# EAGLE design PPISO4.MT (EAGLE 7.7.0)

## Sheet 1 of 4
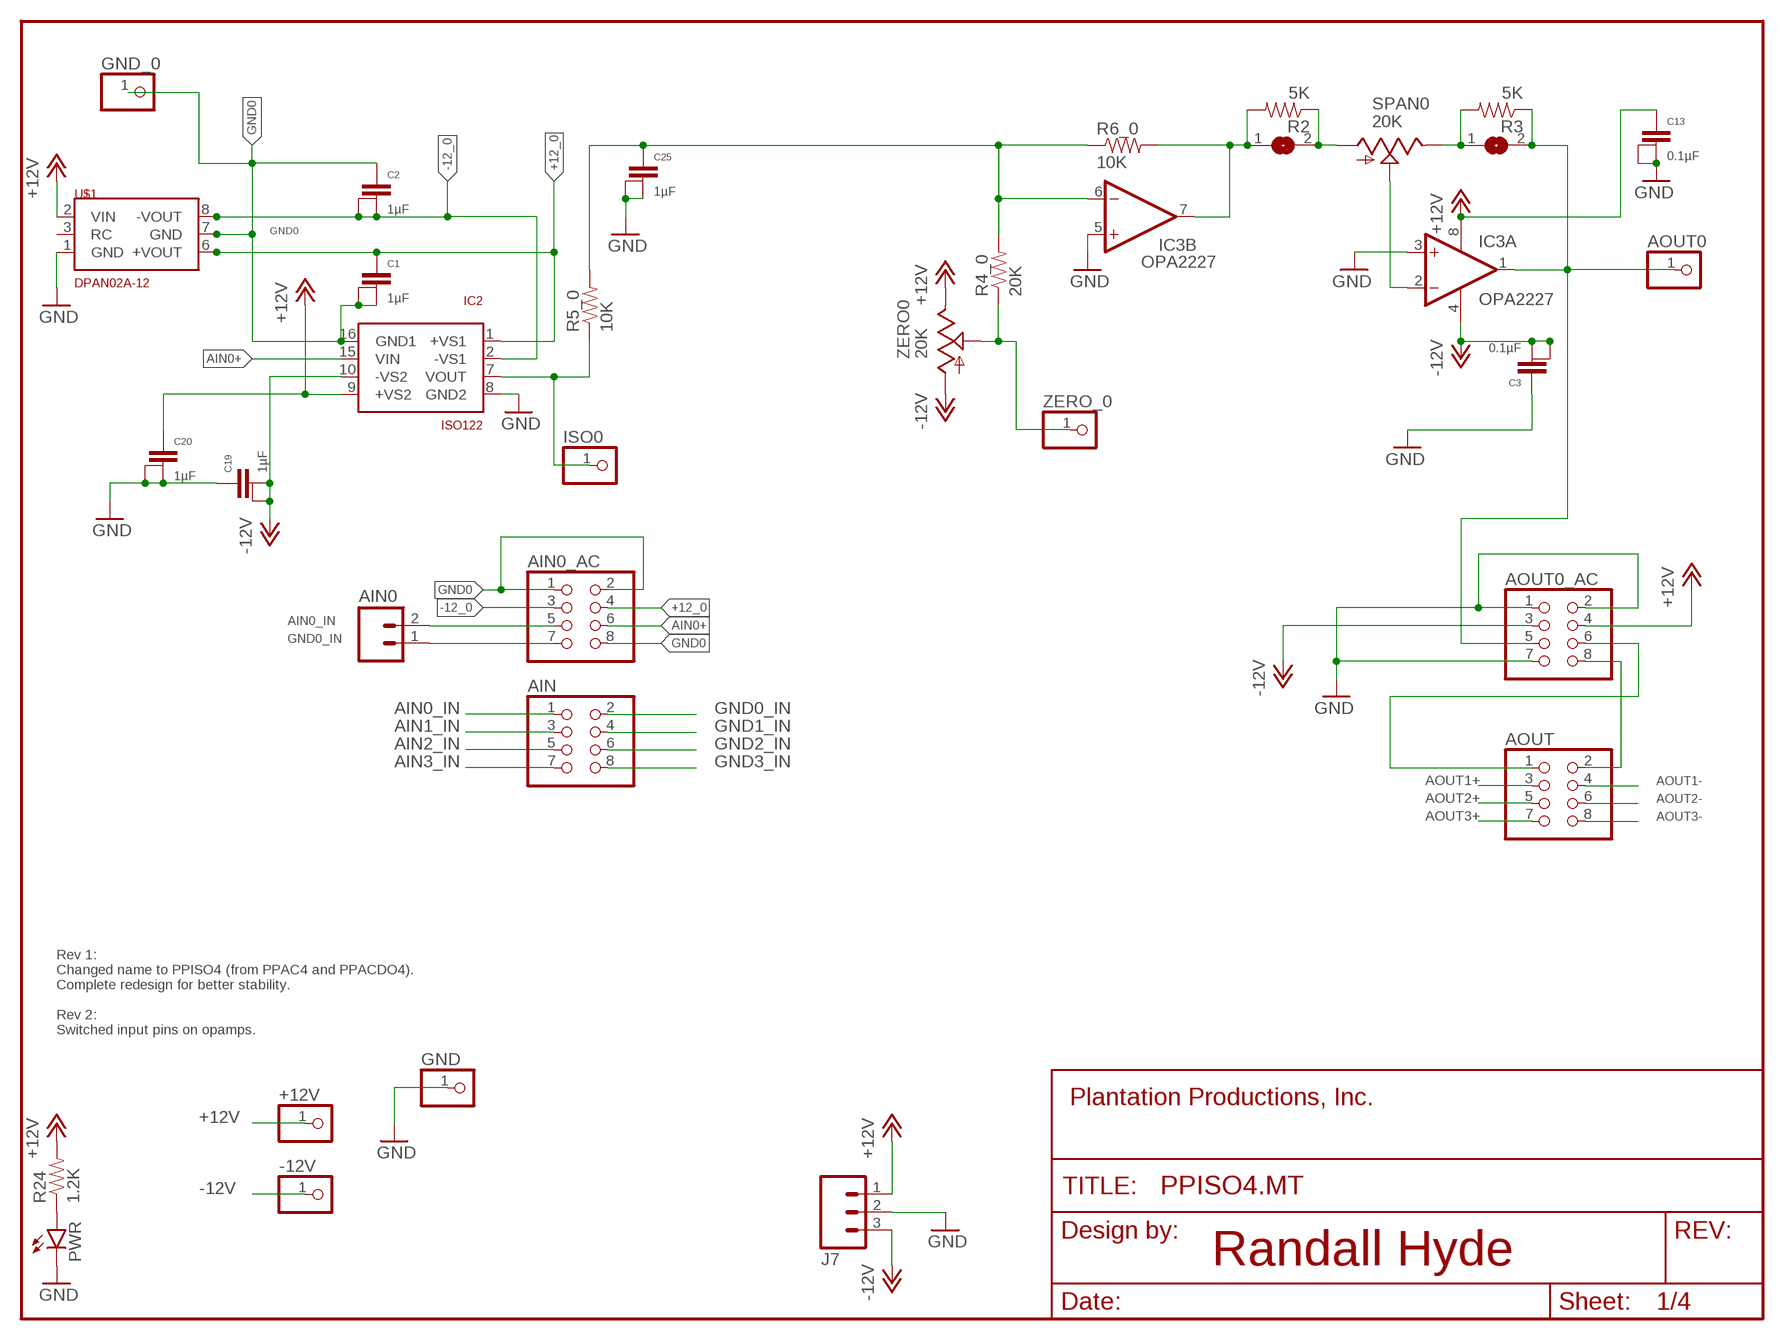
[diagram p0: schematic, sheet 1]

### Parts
+12V  PINHD-1X1  [1X01]
-12V  PINHD-1X1  [1X01]
AIN  PINHD-2X4  [2X04]
AIN0  M025MM  [SCREWTERMINAL-5MM-2]
AIN0_AC  PINHD-2X4  [2X04]
AOUT  PINHD-2X4  [2X04]
AOUT0  PINHD-1X1  [1X01]
AOUT0_AC  PINHD-2X4  [2X04]
C1  1µF  CAPACITOR  [1+2CAP]
C2  1µF  CAPACITOR  [1+2CAP]
C3  0.1µF  CAPACITOR  [1+2CAP]
C13  0.1µF  CAPACITOR  [1+2CAP]
C19  1µF  CAPACITOR  [1+2CAP]
C20  1µF  CAPACITOR  [1+2CAP]
C25  1µF  CAPACITOR  [1+2CAP]
FRAME1  FRAME-LETTERNO_PACKAGE  [DUMMY]
GND  PINHD-1X1  [1X01]
GND_0  PINHD-1X1  [1X01]
IC2  ISO122  [DIL16-8]
IC3  OPA2227  OPA2227N  [DIL08]
ISO0  PINHD-1X1  [1X01]
J7  M03-SCREW-5MM  [SCREWTERMINAL-5MM-3]
PWR  LED5MM  [LED5MM]
R2  5K  10OHM-1/4W-5%(PTH)  [AXIAL-0.3]
R3  5K  10OHM-1/4W-5%(PTH)  [AXIAL-0.3]
R4_0  20K  10OHM-1/4W-5%(PTH)  [AXIAL-0.3]
R5_0  10K  10OHM-1/4W-5%(PTH)  [AXIAL-0.3]
R6_0  10K  10OHM-1/4W-5%(PTH)  [AXIAL-0.3]
R24  1.2K  1KOHM-1/4W-1%(PTH)  [AXIAL-0.3]
SJ3  SOLDERJUMPERCLOSED  [SOLDERJUMPER_CLOSEDWIRE]
SJ4  SOLDERJUMPERCLOSED  [SOLDERJUMPER_CLOSEDWIRE]
SPAN0  20K  MULTIPOT  [B64WY]
U$1  DPAN02E-12  [DPAN-02E-12]
ZERO0  20K  MULTIPOT  [B64WY]
ZERO_0  PINHD-1X1  [1X01]

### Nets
+12_0 [RelayConn]: AIN0_AC.4 C1.1 IC2.1(+VS1) U$1.6(+VOUT)
+12V [RelayConn]: +12V.1 AOUT0_AC.4 C13.1 C20.1 IC2.9(+VS2) IC3.8(P:V+) J7.1 R24.P$2 U$1.2(VIN) ZERO0.E ZERO0.E1(E) ; also sheet 2,3,4
+12V3: R3.P$2 SJ4.1 SPAN0.E SPAN0.E1(E)
-12_0 [RelayConn]: AIN0_AC.3 C2.2@1 C2.2@2 IC2.2(-VS1) U$1.8(-VOUT)
-12V [RelayConn]: -12V.1 AOUT0_AC.3 C3.2@1 C3.2@2 C19.2@1 C19.2@2 IC2.10(-VS2) IC3.4(P:V-) J7.3 ZERO0.A ; also sheet 2,3,4
AIN0+: AIN0_AC.6 IC2.15(VIN)
AIN0_IN: AIN0.2 AIN0_AC.5 AIN.1
AIN1_IN: AIN.3 ; also sheet 2
AIN2_IN: AIN.5 ; also sheet 3
AIN3_IN: AIN.7 ; also sheet 4
AOUT0: AOUT0.1 AOUT0_AC.5 IC3.1(A:OUT) R3.P$1 SJ4.2
AOUT0+: AOUT0_AC.6 AOUT.1
AOUT0-: AOUT0_AC.8 AOUT.2
AOUT1+: AOUT.3 ; also sheet 2
AOUT1-: AOUT.4 ; also sheet 2
AOUT2+: AOUT.5 ; also sheet 3
AOUT2-: AOUT.6 ; also sheet 3
AOUT3+: AOUT.7 ; also sheet 4
AOUT3-: AOUT.8
GND [Ground]: AOUT0_AC.1 AOUT0_AC.2 AOUT0_AC.7 C3.1 C13.2@1 C13.2@2 C19.1 C20.2@1 C20.2@2 C25.2@1 C25.2@2 GND.1 IC2.8(GND2) IC3.3(A:+IN) IC3.5(B:+IN) J7.2 PWR.K(C) U$1.1(GND) ; also sheet 2,3,4
GND0: AIN0_AC.1 AIN0_AC.2 AIN0_AC.8 C1.2@1 C1.2@2 C2.1 GND_0.1 IC2.16(GND1) U$1.7(GND)
GND0_IN: AIN0.1 AIN0_AC.7 AIN.2
GND1_IN: AIN.4 ; also sheet 2
GND2_IN: AIN.6 ; also sheet 3
GND3_IN: AIN.8 ; also sheet 4
IC1_9: IC3.7(B:OUT) R2.P$2 R6_0.P$2 SJ3.1
N$4: IC3.2(A:-IN) SPAN0.A1(S) SPAN0.S SPAN0.S1(S)
N$6: R4_0.P$1 ZERO0.A1(S) ZERO0.S ZERO0.S1(S) ZERO_0.1
N$8: IC2.7(VOUT) ISO0.1 R5_0.P$1
N$26: PWR.A R24.P$1
N$43: C25.1 IC3.6(B:-IN) R4_0.P$2 R5_0.P$2 R6_0.P$1
N$58: R2.P$1 SJ3.2 SPAN0.A
Unconnected: U$1.3(RC)

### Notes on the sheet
- Rev 1:
  Changed name to PPISO4 (from PPAC4 and PPACDO4).
  Complete redesign for better stability.
  
  Rev 2:
  Switched input pins on opamps.
- Randall Hyde

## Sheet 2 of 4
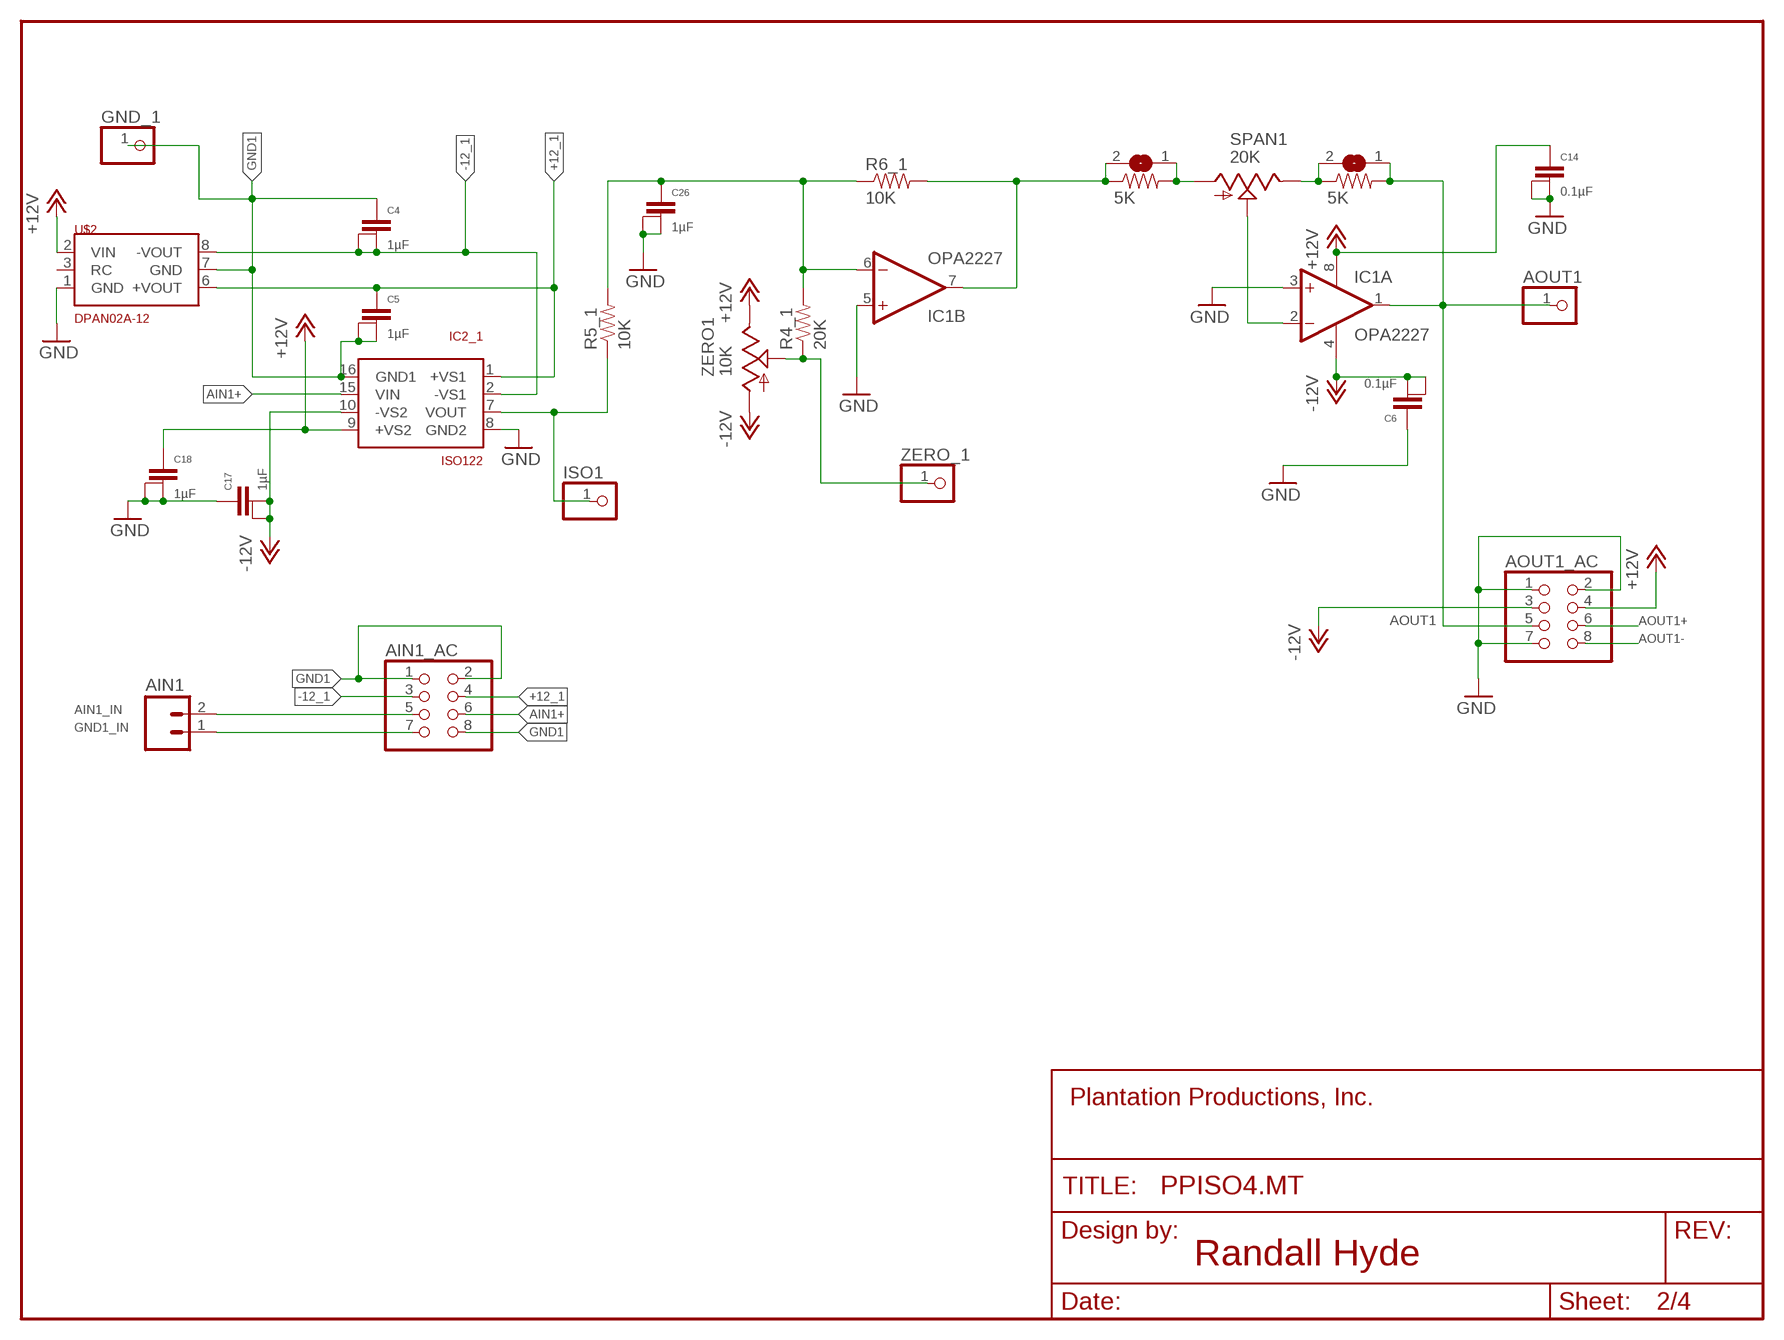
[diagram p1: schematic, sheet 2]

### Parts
AIN1  M025MM  [SCREWTERMINAL-5MM-2]
AIN1_AC  PINHD-2X4  [2X04]
AOUT1  PINHD-1X1  [1X01]
AOUT1_AC  PINHD-2X4  [2X04]
C4  1µF  CAPACITOR  [1+2CAP]
C5  1µF  CAPACITOR  [1+2CAP]
C6  0.1µF  CAPACITOR  [1+2CAP]
C14  0.1µF  CAPACITOR  [1+2CAP]
C17  1µF  CAPACITOR  [1+2CAP]
C18  1µF  CAPACITOR  [1+2CAP]
C26  1µF  CAPACITOR  [1+2CAP]
FRAME2  FRAME-LETTERNO_PACKAGE  [DUMMY]
GND_1  PINHD-1X1  [1X01]
IC1  OPA2227  OPA2227N  [DIL08]
IC2_1  ISO122  [DIL16-8]
ISO1  PINHD-1X1  [1X01]
R4_1  20K  10OHM-1/4W-5%(PTH)  [AXIAL-0.3]
R5_1  10K  10OHM-1/4W-5%(PTH)  [AXIAL-0.3]
R6  5K  10OHM-1/4W-5%(PTH)  [AXIAL-0.3]
R6_1  10K  10OHM-1/4W-5%(PTH)  [AXIAL-0.3]
R11  5K  10OHM-1/4W-5%(PTH)  [AXIAL-0.3]
SJ7  SOLDERJUMPERCLOSED  [SOLDERJUMPER_CLOSEDWIRE]
SJ12  SOLDERJUMPERCLOSED  [SOLDERJUMPER_CLOSEDWIRE]
SPAN1  20K  MULTIPOT  [B64WY]
U$2  DPAN02E-12  [DPAN-02E-12]
ZERO1  10K  MULTIPOT  [B64WY]
ZERO_1  PINHD-1X1  [1X01]

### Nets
+12_1 [RelayConn]: AIN1_AC.4 C5.1 IC2_1.1(+VS1) U$2.6(+VOUT)
+12V [RelayConn]: AOUT1_AC.4 C14.1 C18.1 IC1.8(P:V+) IC2_1.9(+VS2) U$2.2(VIN) ZERO1.E ZERO1.E1(E) ; also sheet 1,3,4
-12_1 [RelayConn]: AIN1_AC.3 C4.2@1 C4.2@2 IC2_1.2(-VS1) U$2.8(-VOUT)
-12V [RelayConn]: AOUT1_AC.3 C6.2@1 C6.2@2 C17.2@1 C17.2@2 IC1.4(P:V-) IC2_1.10(-VS2) ZERO1.A ; also sheet 1,3,4
AIN1+: AIN1_AC.6 IC2_1.15(VIN)
AIN1_IN: AIN1.2 AIN1_AC.5 ; also sheet 1
AOUT1: AOUT1.1 AOUT1_AC.5 IC1.1(A:OUT) R6.P$2 SJ7.1
AOUT1+: AOUT1_AC.6 ; also sheet 1
AOUT1-: AOUT1_AC.8 ; also sheet 1
GND [Ground]: AOUT1_AC.1 AOUT1_AC.2 AOUT1_AC.7 C6.1 C14.2@1 C14.2@2 C17.1 C18.2@1 C18.2@2 C26.2@1 C26.2@2 IC1.3(A:+IN) IC1.5(B:+IN) IC2_1.8(GND2) U$2.1(GND) ; also sheet 1,3,4
GND1: AIN1_AC.1 AIN1_AC.2 AIN1_AC.8 C4.1 C5.2@1 C5.2@2 GND_1.1 IC2_1.16(GND1) U$2.7(GND)
GND1_IN: AIN1.1 AIN1_AC.7 ; also sheet 1
IC2_8: IC1.7(B:OUT) R6_1.P$2 R11.P$1 SJ12.2
N$1: C26.1 IC1.6(B:-IN) R4_1.P$2 R5_1.P$2 R6_1.P$1
N$3: R6.P$1 SJ7.2 SPAN1.E SPAN1.E1(E)
N$19: IC1.2(A:-IN) SPAN1.A1(S) SPAN1.S SPAN1.S1(S)
N$22: IC2_1.7(VOUT) ISO1.1 R5_1.P$1
N$23: R4_1.P$1 ZERO1.A1(S) ZERO1.S ZERO1.S1(S) ZERO_1.1
SPAN1L: R11.P$2 SJ12.1 SPAN1.A
Unconnected: U$2.3(RC)

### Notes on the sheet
- Randall Hyde

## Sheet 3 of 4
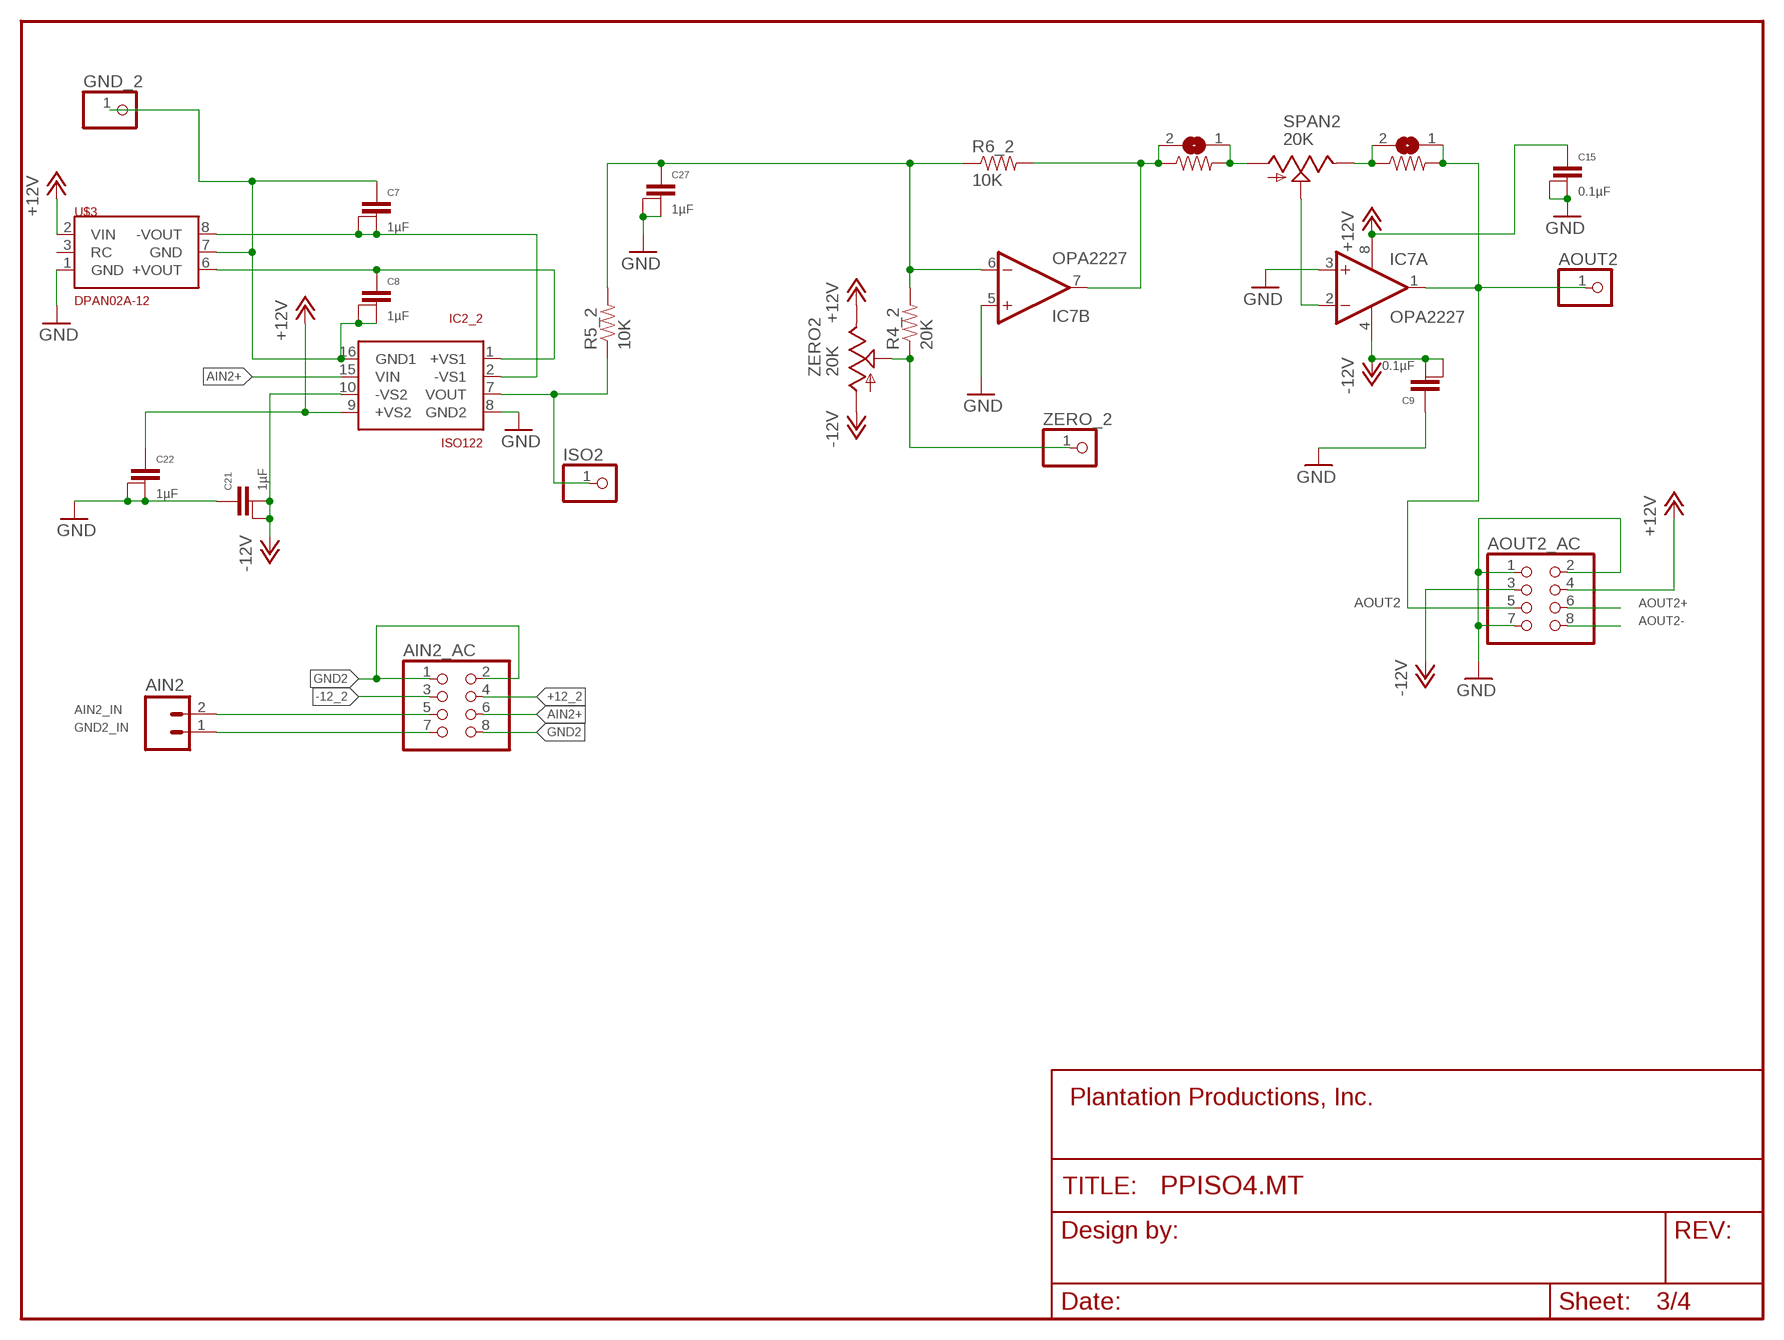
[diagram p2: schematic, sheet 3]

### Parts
AIN2  M025MM  [SCREWTERMINAL-5MM-2]
AIN2_AC  PINHD-2X4  [2X04]
AOUT2  PINHD-1X1  [1X01]
AOUT2_AC  PINHD-2X4  [2X04]
C7  1µF  CAPACITOR  [1+2CAP]
C8  1µF  CAPACITOR  [1+2CAP]
C9  0.1µF  CAPACITOR  [1+2CAP]
C15  0.1µF  CAPACITOR  [1+2CAP]
C21  1µF  CAPACITOR  [1+2CAP]
C22  1µF  CAPACITOR  [1+2CAP]
C27  1µF  CAPACITOR  [1+2CAP]
FRAME3  FRAME-LETTERNO_PACKAGE  [DUMMY]
GND_2  PINHD-1X1  [1X01]
IC2_2  ISO122  [DIL16-8]
IC7  OPA2227  OPA2227N  [DIL08]
ISO2  PINHD-1X1  [1X01]
R4_2  20K  10OHM-1/4W-5%(PTH)  [AXIAL-0.3]
R5_2  10K  10OHM-1/4W-5%(PTH)  [AXIAL-0.3]
R6_2  10K  10OHM-1/4W-5%(PTH)  [AXIAL-0.3]
R12  5K  10OHM-1/4W-5%(PTH)  [AXIAL-0.3]
R17  5K  10OHM-1/4W-5%(PTH)  [AXIAL-0.3]
SJ13  SOLDERJUMPERCLOSED  [SOLDERJUMPER_CLOSEDWIRE]
SJ18  SOLDERJUMPERCLOSED  [SOLDERJUMPER_CLOSEDWIRE]
SPAN2  20K  MULTIPOT  [B64WY]
U$3  DPAN02E-12  [DPAN-02E-12]
ZERO2  20K  MULTIPOT  [B64WY]
ZERO_2  PINHD-1X1  [1X01]

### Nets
+12_2 [RelayConn]: AIN2_AC.4 C8.1 IC2_2.1(+VS1) U$3.6(+VOUT)
+12V [RelayConn]: AOUT2_AC.4 C15.1 C22.1 IC2_2.9(+VS2) IC7.8(P:V+) U$3.2(VIN) ZERO2.E ZERO2.E1(E) ; also sheet 1,2,4
+12V10: R17.P$2 SJ18.1 SPAN2.A
-12_2 [RelayConn]: AIN2_AC.3 C7.2@1 C7.2@2 IC2_2.2(-VS1) U$3.8(-VOUT)
-12V [RelayConn]: AOUT2_AC.3 C9.2@1 C9.2@2 C21.2@1 C21.2@2 IC2_2.10(-VS2) IC7.4(P:V-) ZERO2.A ; also sheet 1,2,4
AIN2+: AIN2_AC.6 IC2_2.15(VIN)
AIN2_IN: AIN2.2 AIN2_AC.5 ; also sheet 1
AOUT2: AOUT2.1 AOUT2_AC.5 IC7.1(A:OUT) R12.P$2 SJ13.1
AOUT2+: AOUT2_AC.6 ; also sheet 1
AOUT2-: AOUT2_AC.8 ; also sheet 1
GND [Ground]: AOUT2_AC.1 AOUT2_AC.2 AOUT2_AC.7 C9.1 C15.2@1 C15.2@2 C21.1 C22.2@1 C22.2@2 C27.2@1 C27.2@2 IC2_2.8(GND2) IC7.3(A:+IN) IC7.5(B:+IN) U$3.1(GND) ; also sheet 1,2,4
GND2: AIN2_AC.1 AIN2_AC.2 AIN2_AC.8 C7.1 C8.2@1 C8.2@2 GND_2.1 IC2_2.16(GND1) U$3.7(GND)
GND2_IN: AIN2.1 AIN2_AC.7 ; also sheet 1
N$18: R12.P$1 SJ13.2 SPAN2.E SPAN2.E1(E)
N$34: IC2_2.7(VOUT) ISO2.1 R5_2.P$1
N$35: IC7.2(A:-IN) SPAN2.A1(S) SPAN2.S SPAN2.S1(S)
N$36: IC7.7(B:OUT) R6_2.P$2 R17.P$1 SJ18.2
N$40: R4_2.P$1 ZERO2.A1(S) ZERO2.S ZERO2.S1(S) ZERO_2.1
N$60: C27.1 IC7.6(B:-IN) R4_2.P$2 R5_2.P$2 R6_2.P$1
Unconnected: U$3.3(RC)

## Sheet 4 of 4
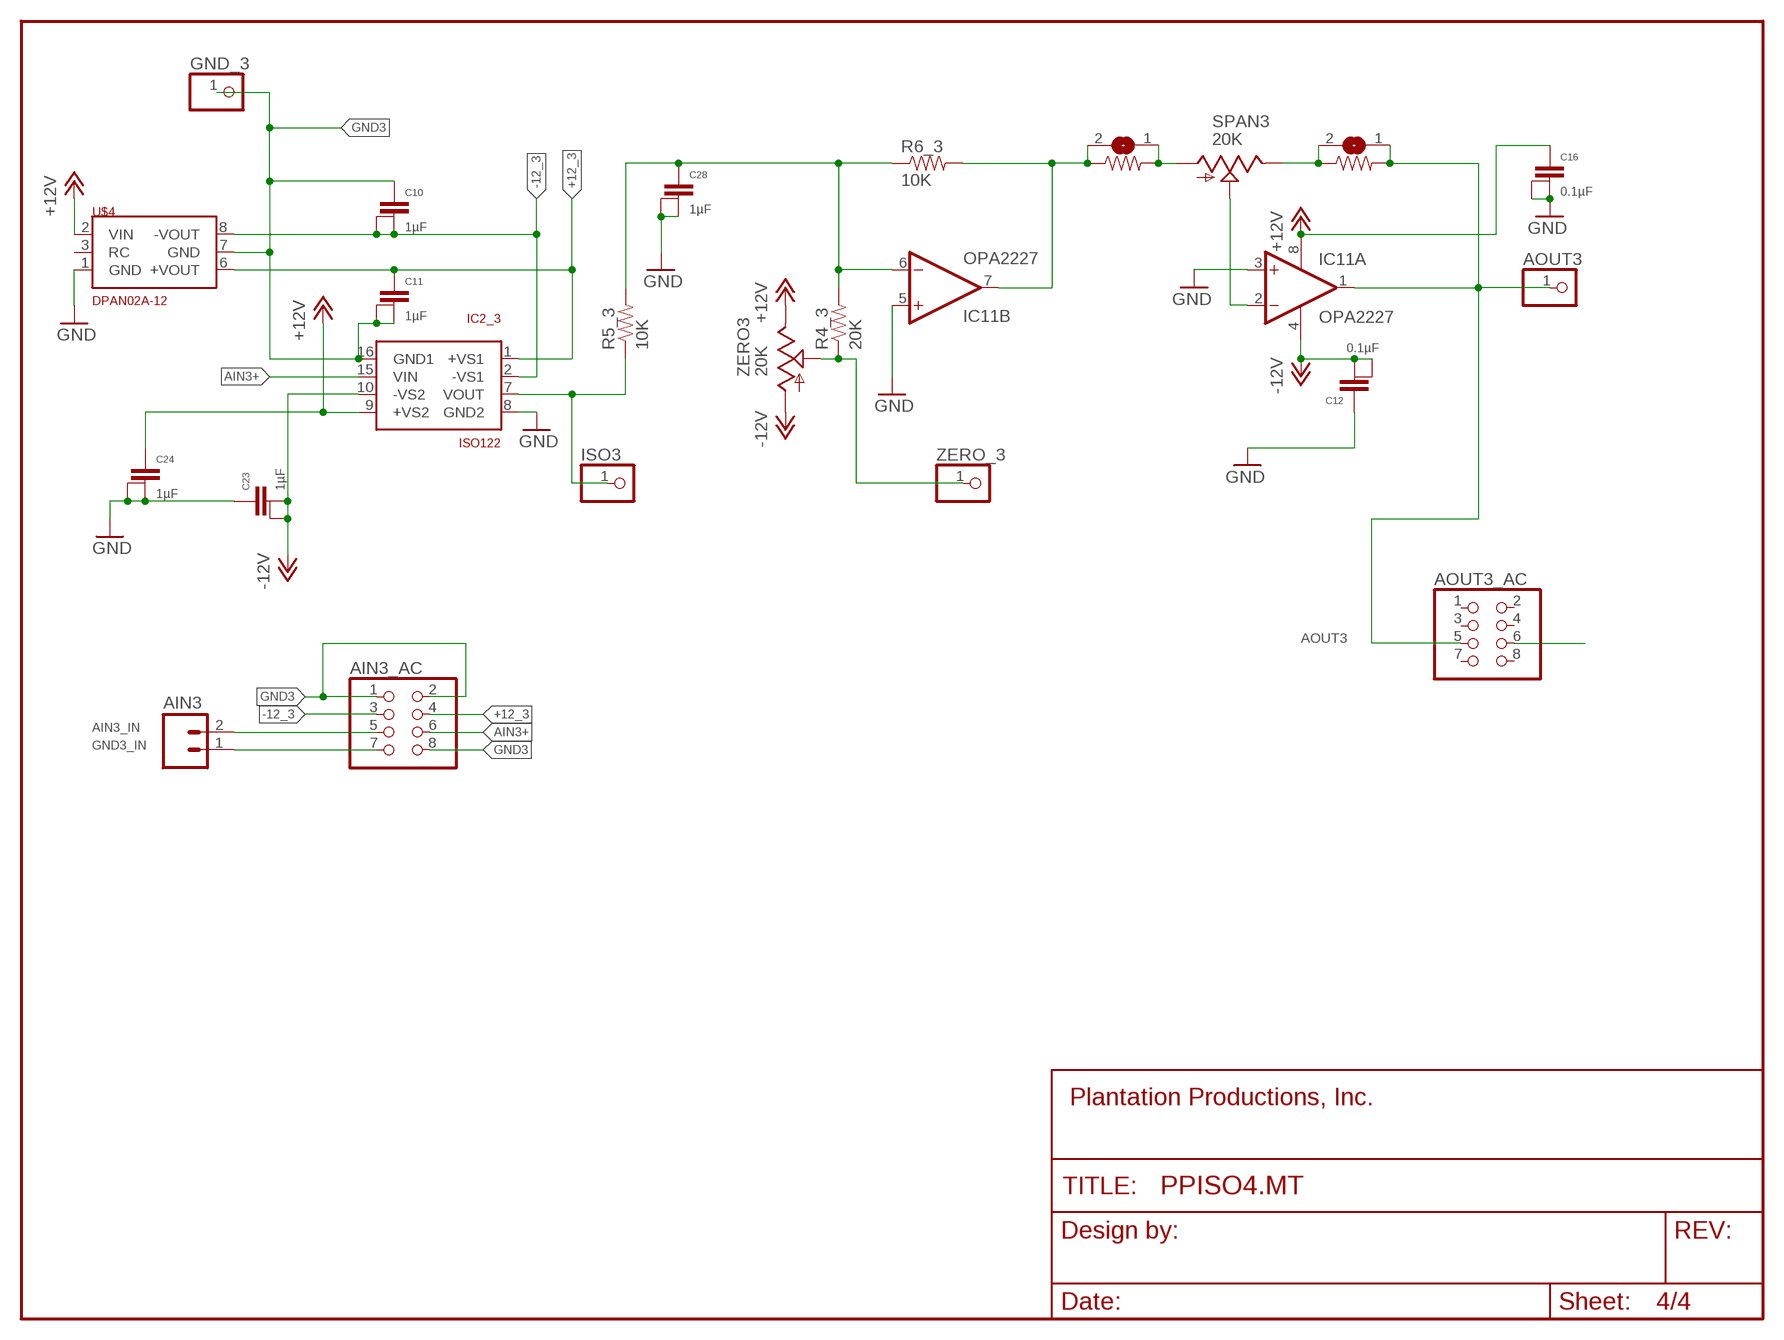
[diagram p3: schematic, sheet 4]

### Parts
AIN3  M025MM  [SCREWTERMINAL-5MM-2]
AIN3_AC  PINHD-2X4  [2X04]
AOUT3  PINHD-1X1  [1X01]
AOUT3_AC  PINHD-2X4  [2X04]
C10  1µF  CAPACITOR  [1+2CAP]
C11  1µF  CAPACITOR  [1+2CAP]
C12  0.1µF  CAPACITOR  [1+2CAP]
C16  0.1µF  CAPACITOR  [1+2CAP]
C23  1µF  CAPACITOR  [1+2CAP]
C24  1µF  CAPACITOR  [1+2CAP]
C28  1µF  CAPACITOR  [1+2CAP]
FRAME4  FRAME-LETTERNO_PACKAGE  [DUMMY]
GND_3  PINHD-1X1  [1X01]
IC2_3  ISO122  [DIL16-8]
IC11  OPA2227  OPA2227N  [DIL08]
ISO3  PINHD-1X1  [1X01]
R4_3  20K  10OHM-1/4W-5%(PTH)  [AXIAL-0.3]
R5_3  10K  10OHM-1/4W-5%(PTH)  [AXIAL-0.3]
R6_3  10K  10OHM-1/4W-5%(PTH)  [AXIAL-0.3]
R18  5K  10OHM-1/4W-5%(PTH)  [AXIAL-0.3]
R23  5K  10OHM-1/4W-5%(PTH)  [AXIAL-0.3]
SJ19  SOLDERJUMPERCLOSED  [SOLDERJUMPER_CLOSEDWIRE]
SJ24  SOLDERJUMPERCLOSED  [SOLDERJUMPER_CLOSEDWIRE]
SPAN3  20K  MULTIPOT  [B64WY]
U$4  DPAN02E-12  [DPAN-02E-12]
ZERO3  20K  MULTIPOT  [B64WY]
ZERO_3  PINHD-1X1  [1X01]

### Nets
+12_3 [RelayConn]: AIN3_AC.4 C11.1 IC2_3.1(+VS1) U$4.6(+VOUT)
+12V [RelayConn]: C16.1 C24.1 IC2_3.9(+VS2) IC11.8(P:V+) U$4.2(VIN) ZERO3.E ZERO3.E1(E) ; also sheet 1,2,3
+12V4: R18.P$2 SJ19.1 SPAN3.A
-12_3 [RelayConn]: AIN3_AC.3 C10.2@1 C10.2@2 IC2_3.2(-VS1) U$4.8(-VOUT)
-12V [RelayConn]: C12.2@1 C12.2@2 C23.2@1 C23.2@2 IC2_3.10(-VS2) IC11.4(P:V-) ZERO3.A ; also sheet 1,2,3
AIN3+: AIN3_AC.6 IC2_3.15(VIN)
AIN3_IN: AIN3.2 AIN3_AC.5 ; also sheet 1
AOUT3: AOUT3.1 AOUT3_AC.5 IC11.1(A:OUT) R23.P$2 SJ24.1
AOUT3+: AOUT3_AC.6 ; also sheet 1
GND [Ground]: C12.1 C16.2@1 C16.2@2 C23.1 C24.2@1 C24.2@2 C28.2@1 C28.2@2 IC2_3.8(GND2) IC11.3(A:+IN) IC11.5(B:+IN) U$4.1(GND) ; also sheet 1,2,3
GND3: AIN3_AC.1 AIN3_AC.2 AIN3_AC.8 C10.1 C11.2@1 C11.2@2 GND_3.1 IC2_3.16(GND1) U$4.7(GND)
GND3_IN: AIN3.1 AIN3_AC.7 ; also sheet 1
N$17: IC11.2(A:-IN) SPAN3.A1(S) SPAN3.S SPAN3.S1(S)
N$27: IC11.7(B:OUT) R6_3.P$2 R18.P$1 SJ19.2
N$37: R23.P$1 SJ24.2 SPAN3.E SPAN3.E1(E)
N$39: C28.1 IC11.6(B:-IN) R4_3.P$2 R5_3.P$2 R6_3.P$1
N$55: IC2_3.7(VOUT) ISO3.1 R5_3.P$1
N$56: R4_3.P$1 ZERO3.A1(S) ZERO3.S ZERO3.S1(S) ZERO_3.1
Unconnected: AOUT3_AC.1 AOUT3_AC.2 AOUT3_AC.3 AOUT3_AC.4 AOUT3_AC.7 AOUT3_AC.8 U$4.3(RC)

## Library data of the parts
+12V -12V AOUT0 AOUT1-AOUT3 GND GND_0 GND_1-GND_3 ISO0 ISO1-ISO3 ZERO_0 ZERO_1-ZERO_3 = pinhead:PINHD-1X1: PIN HEADER
AIN AIN0_AC AIN1_AC AIN2_AC AIN3_AC AOUT AOUT0_AC AOUT1_AC AOUT2_AC AOUT3_AC = pinhead:PINHD-2X4: PIN HEADER
AIN0 AIN1-AIN3 = SparkFun-Connectors:M02: Standard 2-pin 0.1" header. Use with; STOREFRONT_ID: PRT-08432
C1-C28 = PlantProd:CAPACITOR: Capacitor with three terminals to support multiple capacitor sizes.
FRAME1-FRAME4 = SparkFun-Aesthetics:FRAME-LETTER: Schematic Frame; DESIGNER: Nobody; VERSION: v01
IC1 IC3 IC7 IC11 = linear:OPA222*: High Precision, Low Noise OPERATIONAL AMPLIFIERS Source: http://focus.ti.com/lit/ds/symlink/opa227.pdf
IC2 IC2_1-IC2_3 = PlantProd:ISO122: ISO122 - single channel isolation amplifier
J7 = SparkFun-Connectors:M03: Header 3 Standard 3-pin 0.1" header. Use with straight break away headers (SKU : PRT-00116), right angle break away headers (PRT-00553), swiss pins (PRT-00743), machine pins (PRT-00117), and female headers (PRT-00115). Molex polarized connector foot print use with SKU : PRT-08232 with associated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; STOREFRONT_ID: PRT-08433
PWR = SparkFun-LED:LED: LEDs
R2 R3 R4_0 R4_1-R4_3 R5_0 R5_1-R5_3 R6 R6_0 R6_1-R6_3 R11 R12 R17 R18 R23 = SparkFun-Resistors:10OHM-1/4W-5%(PTH): RES-10698; PROD_ID: RES-10698; VALUE: 10
R24 = SparkFun-Resistors:1KOHM-1/4W-1%(PTH): RES-12182; PROD_ID: RES-12182; VALUE: 1K
SJ3 SJ4 SJ7 SJ12 SJ13 SJ18 SJ19 SJ24 = microbuilder:SOLDERJUMPER: SMD Solder JUMPER
SPAN0 SPAN1-SPAN3 ZERO0 ZERO1-ZERO3 = PlantProd:MULTIPOT
U$1-U$4 = PlantProd:DPAN02E-12

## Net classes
1 Ground: width 0.762 mm, drill 1 mm, clearance 0.102 mm
2 RelayConn: width 1.016 mm, drill 0.025 mm, clearance 0.508 mm
3 HiCurSignal: width 1.016 mm, drill 0.025 mm, clearance 1.016 mm

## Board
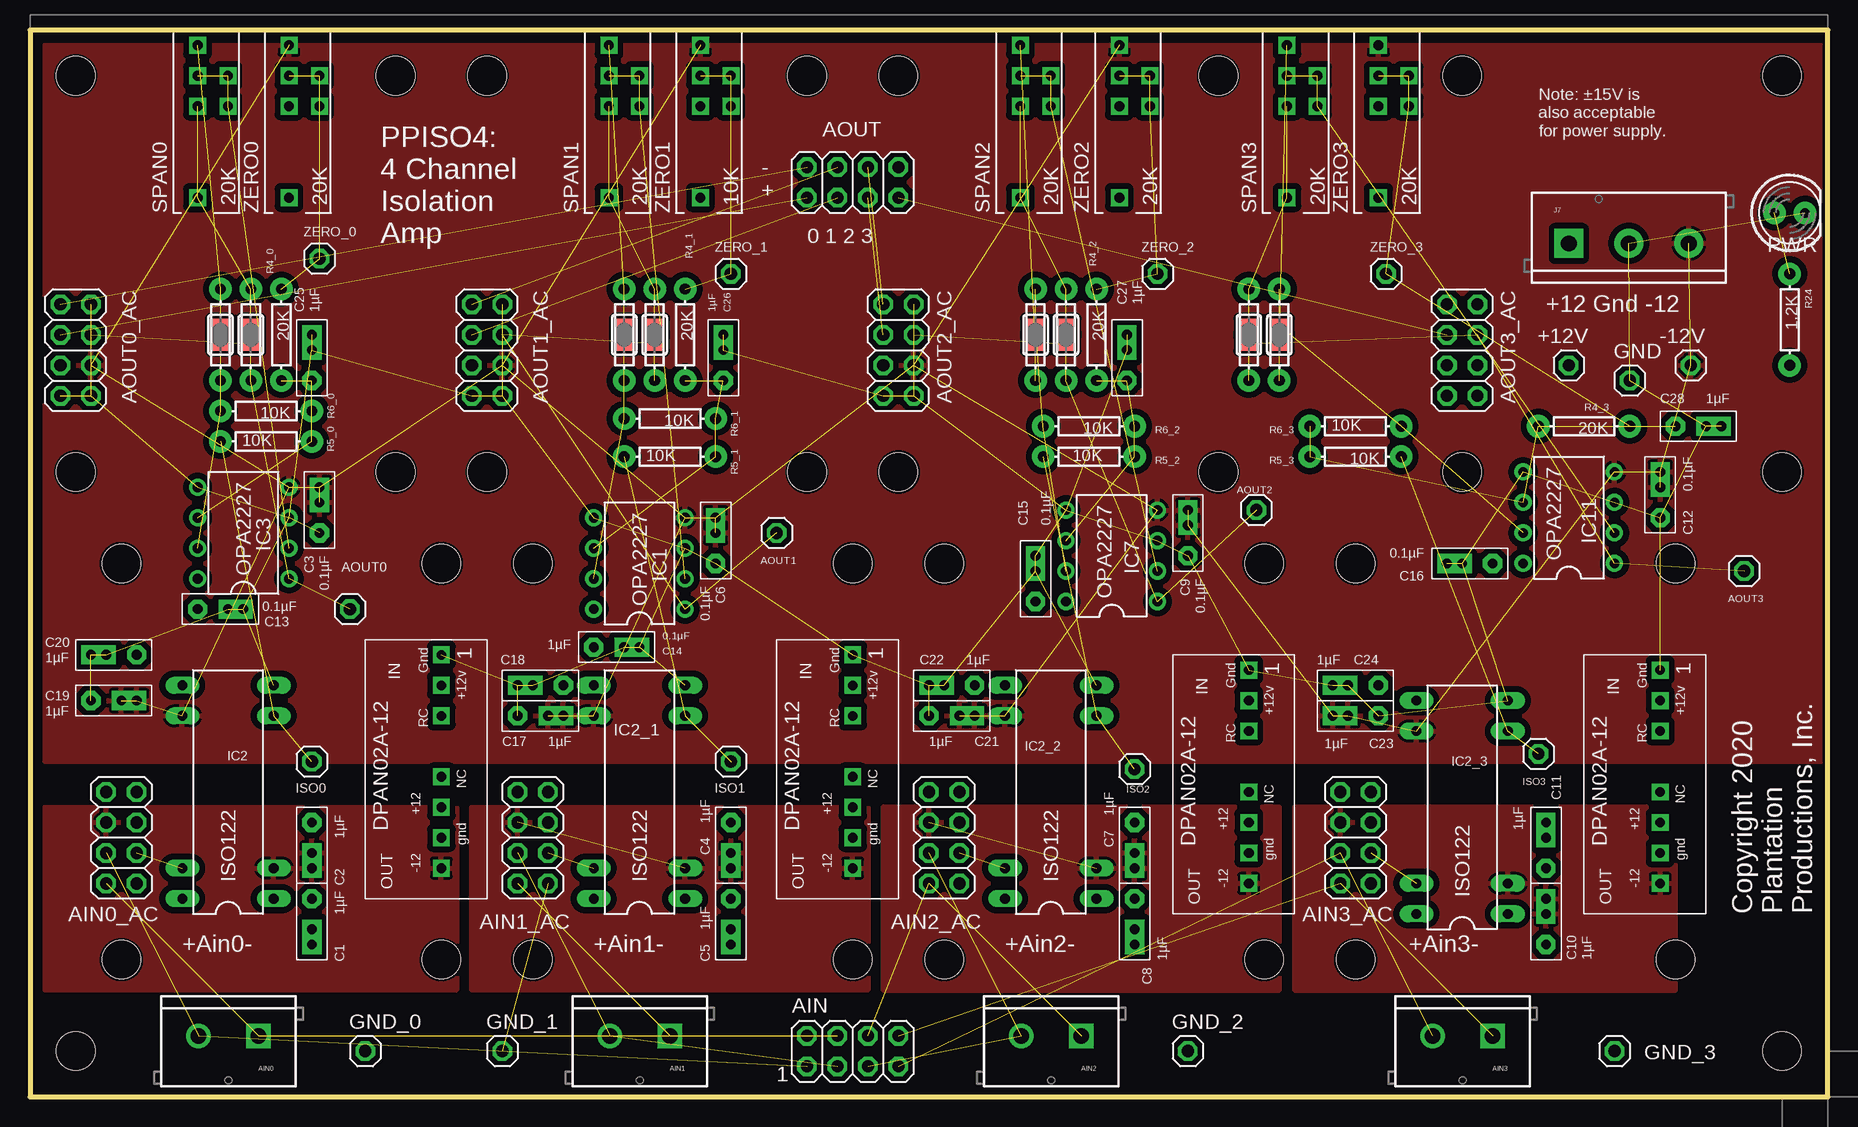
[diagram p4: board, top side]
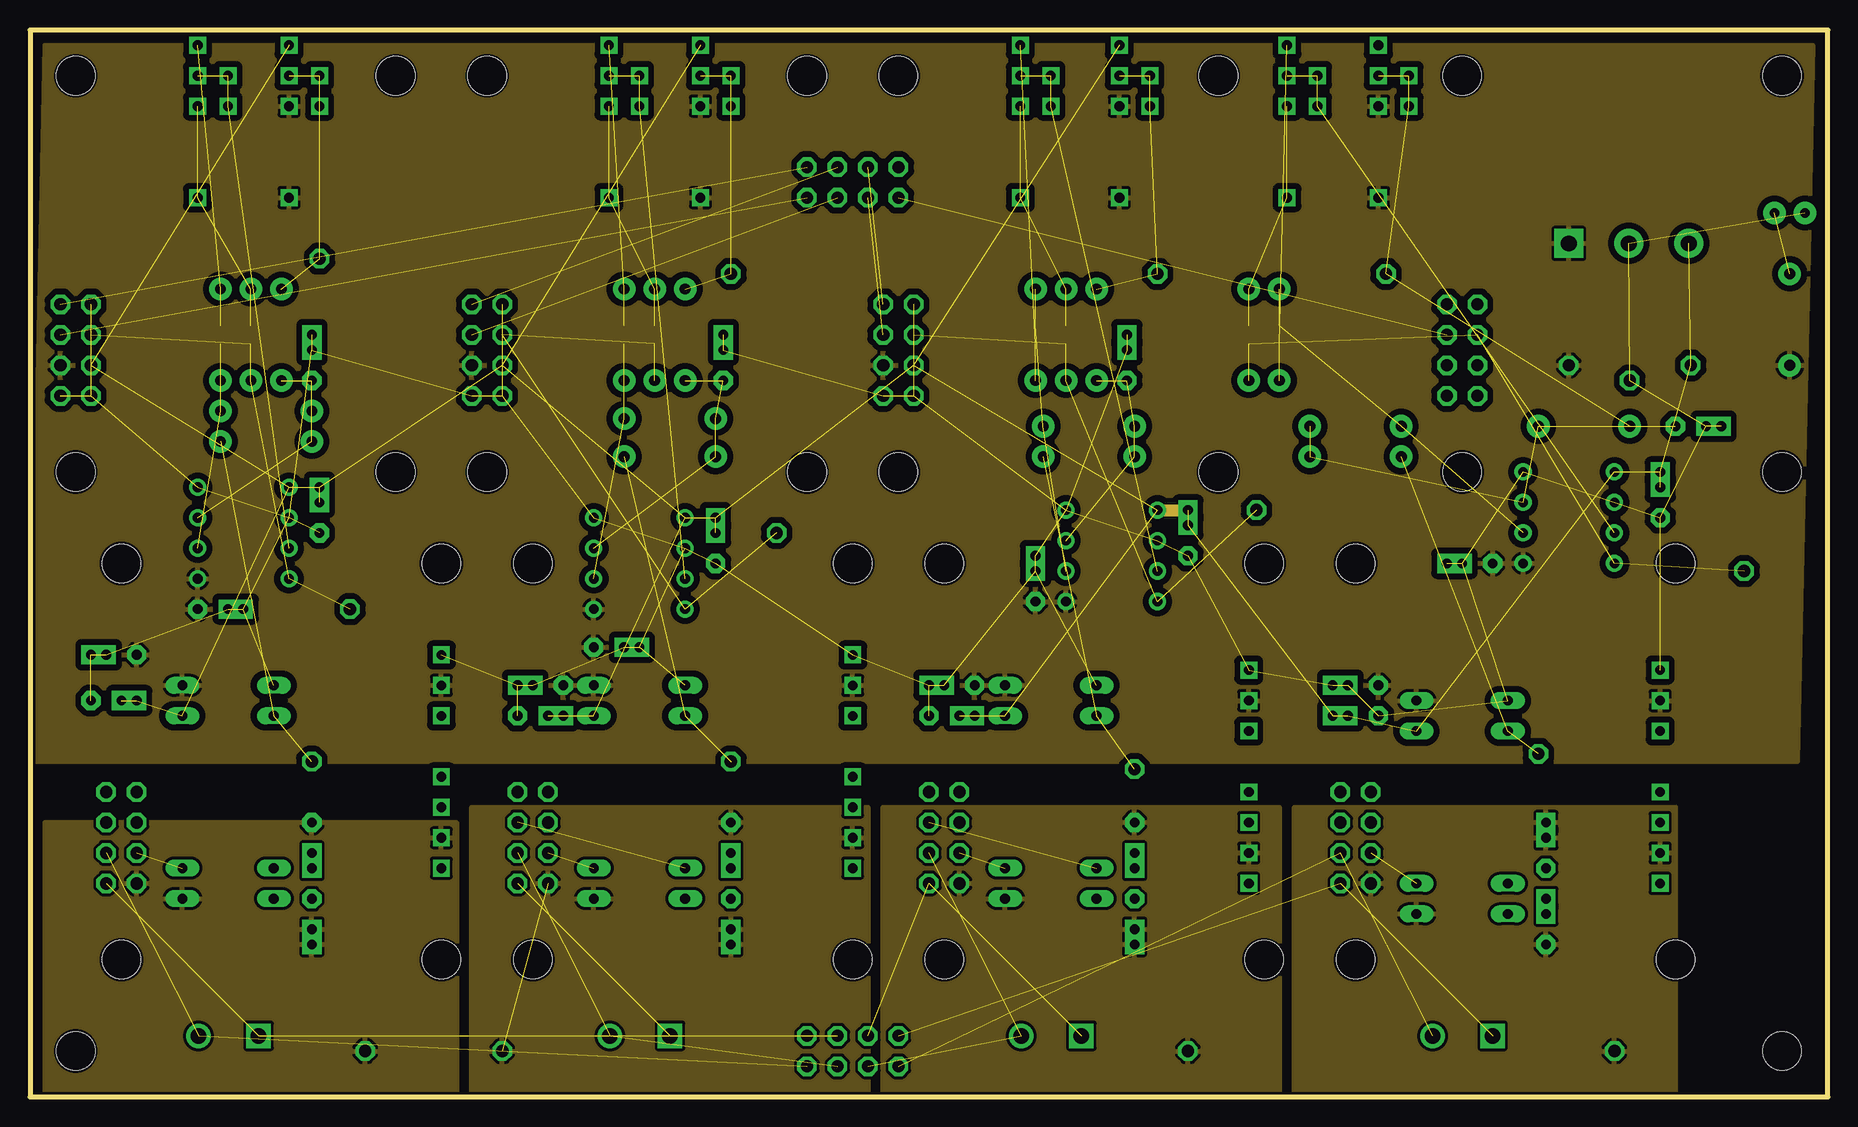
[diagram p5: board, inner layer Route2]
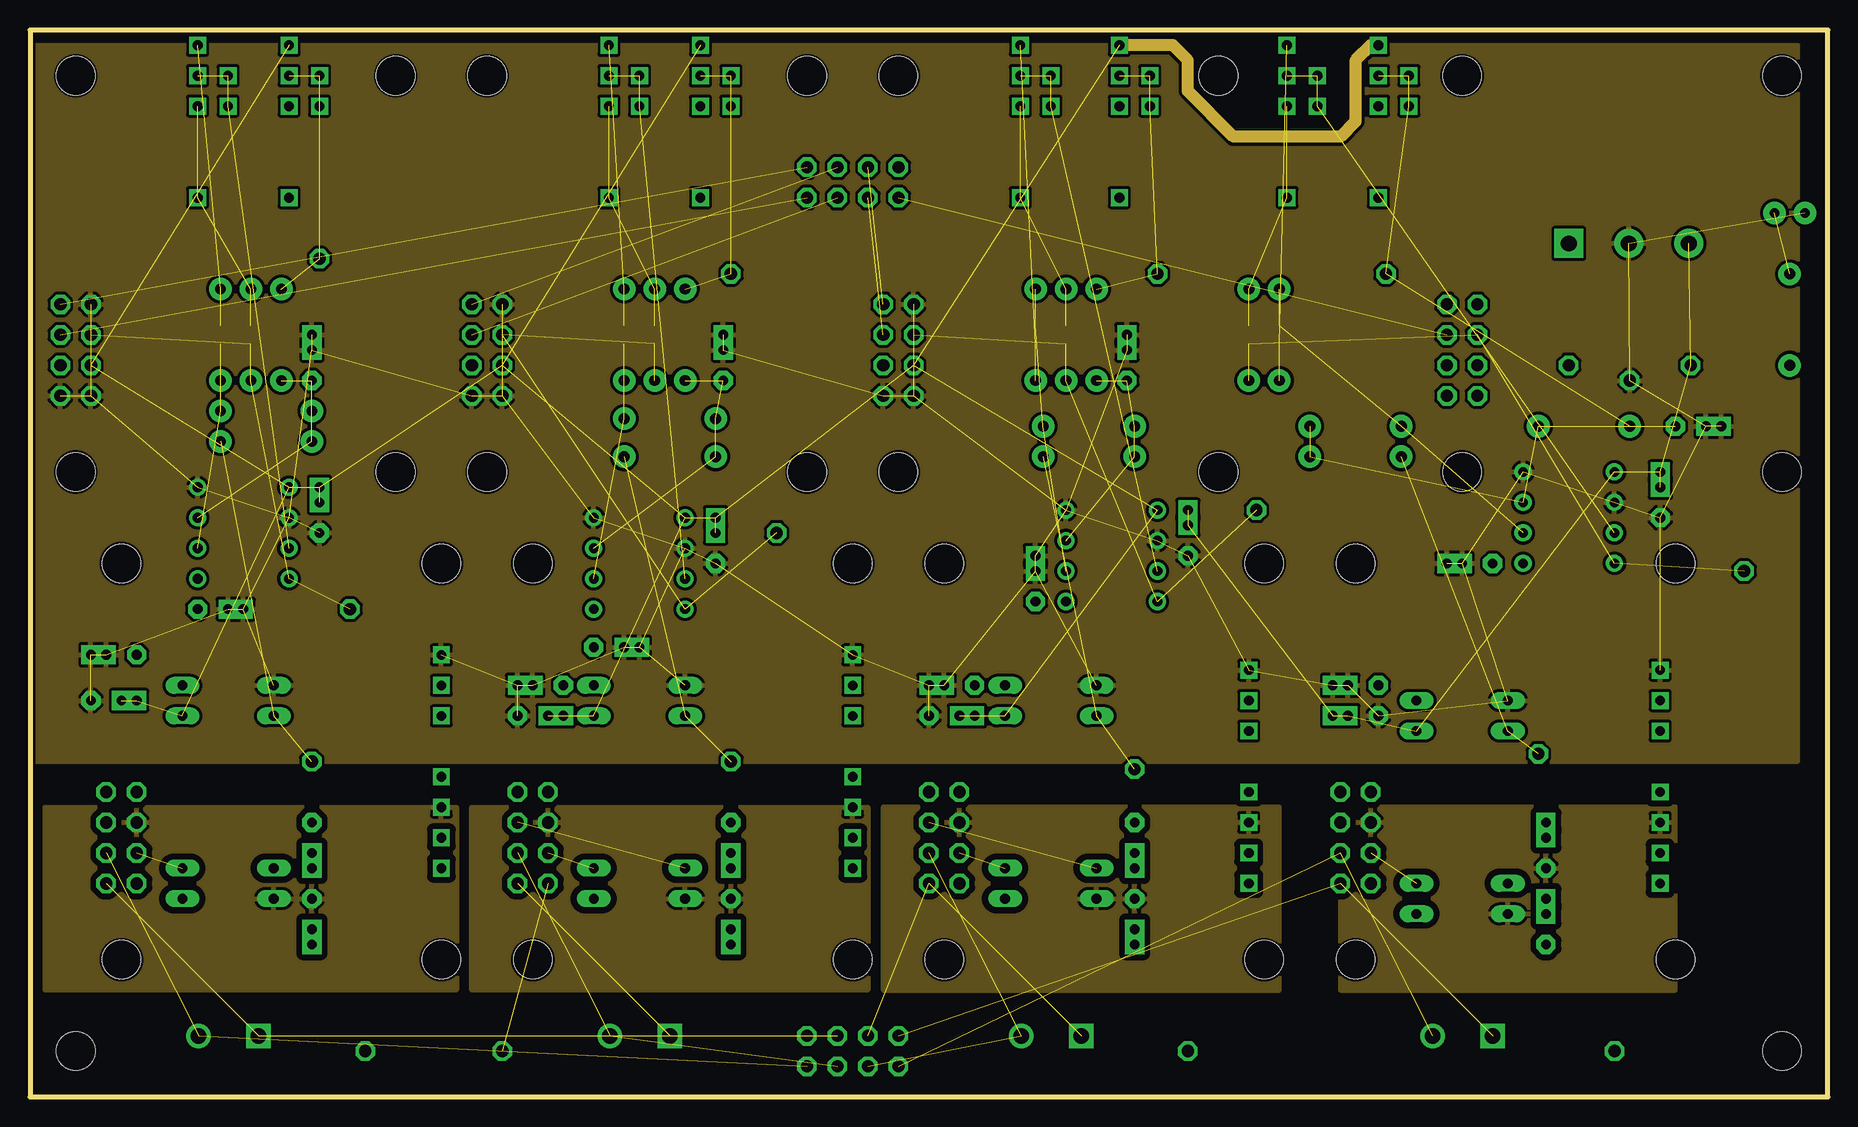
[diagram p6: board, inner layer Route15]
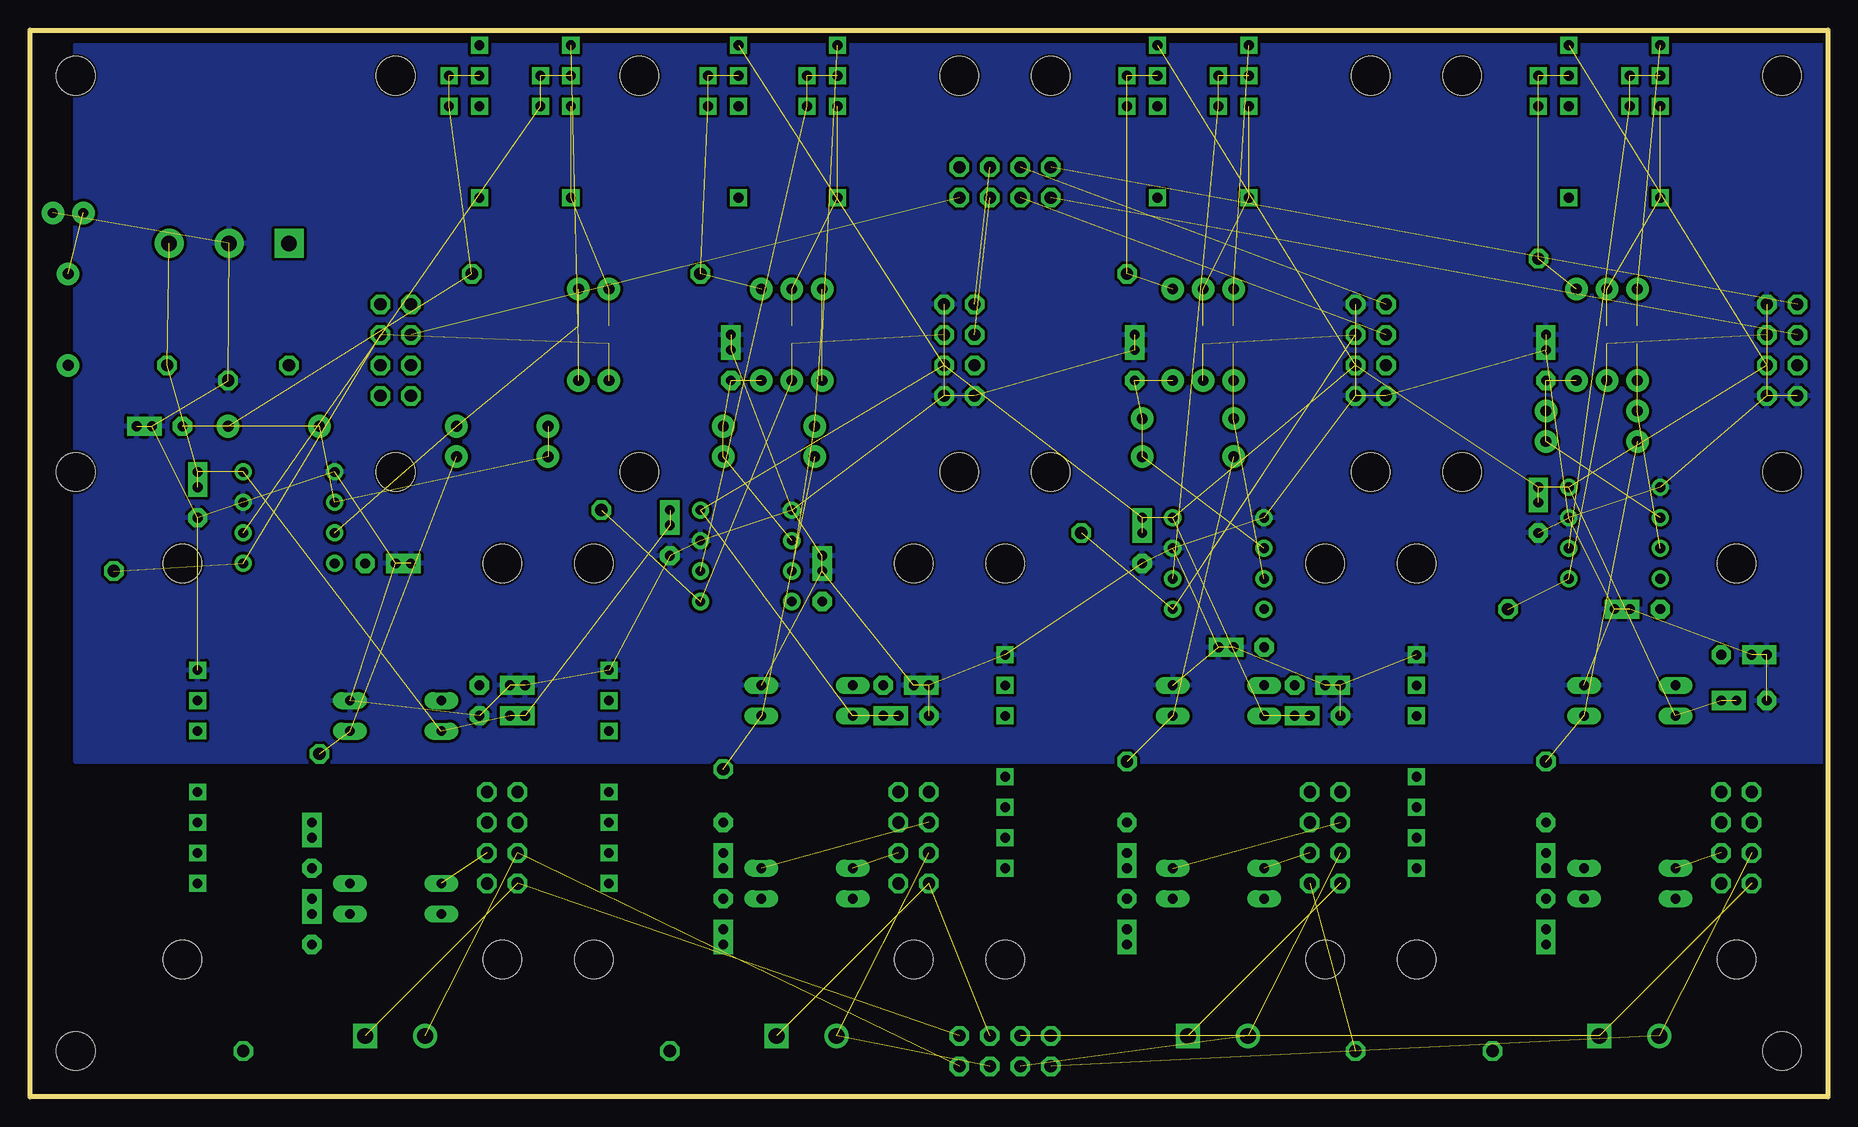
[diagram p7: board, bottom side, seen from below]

Size 149.86 x 88.9 mm. Coordinates in mm from the lower left corner, seen from the top.
Outline: 0,0 149.86,0 149.86,88.9 0,88.9 0,0
Copper layers (1*2*15*16): Top 0.035mm / dielectric 1.5mm / Route2 0.035mm / dielectric 0.15mm / Route15 0.035mm / dielectric 0.2mm / Bottom 0.035mm
Design rules "SeeedStudio_2layer_DRU_no_angle_20140221 *": minimum track width 10mil, minimum drill 20mil, track to track 10mil, track to pad 10mil, pad to pad 10mil, via to via 10mil, smd to smd 8mil, copper to edge 8mil, drill to drill 8mil, minimum pad ring 12mil, minimum via ring 10mil, stop-mask expansion 4mil, vias tented up to drill 25mil, thermal gap 10mil
Holes 3.2 mm at 3.81,85.09 3.81,3.81 146.05,85.09 146.05,3.81 7.62,11.43 7.62,44.45 41.91,11.43 41.91,44.45 76.2,11.43 76.2,44.45 110.49,11.43 110.49,44.45 137.16,44.45 137.16,11.43 3.81,52.07 3.81,85.09 38.1,52.07 38.1,85.09 72.39,85.09 72.39,52.07 99.06,85.09 119.38,52.07 157.48,83.82 146.05,52.07 34.29,44.45 34.29,11.43 68.58,11.43 30.48,85.09 64.77,85.09 64.77,52.07 119.38,85.09 30.48,52.07 99.06,52.07 68.58,44.45 102.87,44.45 102.87,11.43

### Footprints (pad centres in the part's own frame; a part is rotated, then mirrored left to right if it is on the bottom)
1X01 = drill 1.016 octagon: 1 0,0
2X04 = drill 1.016 octagon: 1 -3.81,-1.27; 2 -3.81,1.27; 3 -1.27,-1.27; 4 -1.27,1.27; 5 1.27,-1.27; 6 1.27,1.27; 7 3.81,-1.27; 8 3.81,1.27
SCREWTERMINAL-5MM-2 = drill 1.3 pad 2.032 square: 1 0,0 | drill 1.3 pad 2.032: 2 5,0
1+2CAP = drill 0.813 pad 1.6 octagon: 1 -2.54,0 | drill 0.813 pad 1.6 square: 2@1 0,0; 2@2 1.27,0
DIL08 = drill 0.813 pad 1.27: 1 -3.81,-3.81; 2 -1.27,-3.81; 3 1.27,-3.81; 4 3.81,-3.81; 5 3.81,3.81; 6 1.27,3.81; 7 -1.27,3.81; 8 -3.81,3.81
DIL16-8 = drill 0.813 long: 1 -8.89,-3.81; 2 -6.35,-3.81; 7 6.35,-3.81; 8 8.89,-3.81; 9 8.89,3.81; 10 6.35,3.81; 15 -6.35,3.81; 16 -8.89,3.81
SCREWTERMINAL-5MM-3 = drill 1.3 pad 2.413 square: 1 0,0 | drill 1.3 pad 2.413: 2 5,0; 3 10,0
LED5MM = drill 0.813 pad 1.88: A -1.27,0; K 1.27,0
AXIAL-0.3 = drill 0.9 pad 1.88: P$1 -3.81,0; P$2 3.81,0
SOLDERJUMPER_CLOSEDWIRE = smd 1.168 x 1.6: 1 -0.762,0; 2 0.762,0 | smd 0.635 x 0.203: WIRE 0,0
B64WY = drill 0.813 square: A 2.54,0; A1 0,-2.54; E -2.54,0; E1 -10.16,0; S 0,0; S1 -2.54,-2.54
DPAN-02E-12 = drill 0.8 square: 1 -2.54,2.54; 2 0,2.54; 3 2.54,2.54; 5 7.62,2.54; 6 10.16,2.54; 7 12.7,2.54; 8 15.24,2.54

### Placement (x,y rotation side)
+12V  128.27,60.96 0 top
-12V  138.43,60.96 0 top
AIN  68.58,3.81 0 top
AIN0  19.05,5.08 180 top
AIN0_AC  7.62,21.59 270 top
AIN1  53.34,5.08 180 top
AIN1_AC  41.91,21.59 270 top
AIN2  87.63,5.08 180 top
AIN2_AC  76.2,21.59 270 top
AIN3  121.92,5.08 180 top
AIN3_AC  110.49,21.59 270 top
AOUT  68.58,76.2 0 top
AOUT0  26.67,40.64 0 top
AOUT0_AC  3.81,62.23 90 top
AOUT1  62.23,46.99 0 top
AOUT1_AC  38.1,62.23 90 top
AOUT2  102.23,48.9 180 top
AOUT2_AC  72.39,62.23 90 top
AOUT3  142.88,43.81 0 top
AOUT3_AC  119.38,62.23 90 top
C1  23.5,13.97 270 top
C2  23.5,20.32 270 top
C3  24.13,49.53 90 top
C4  58.42,20.32 270 top
C5  58.42,13.97 270 top
C6  57.15,46.99 90 top
C7  92.08,20.32 270 top
C8  92.08,13.97 270 top
C9  96.52,47.62 90 top
C10  126.36,15.24 90 top
C11  126.36,21.59 90 top
C12  135.89,50.8 90 top
C13  16.51,40.64 0 top
C14  49.53,37.47 0 top
C15  83.82,43.81 90 top
C16  119.38,44.45 180 top
C17  43.18,31.75 0 top
C18  41.91,34.29 180 top
C19  7.62,33.02 0 top
C20  6.35,36.83 180 top
C21  77.47,31.75 0 top
C22  76.2,34.29 180 top
C23  109.86,31.75 180 top
C24  109.86,34.29 180 top
C25  23.5,62.23 90 top
C26  57.78,62.23 90 top
C27  91.44,62.23 90 top
C28  139.7,55.88 0 top
FRAME1  114.3,1.27 0 top
FRAME2  114.3,2.54 90 top
FRAME3  2.54,-2.54 0 top
FRAME4  not placed on the board
GND  133.35,59.69 0 top
GND_0  27.94,3.81 0 top
GND_1  39.37,3.81 0 top
GND_2  96.52,3.81 0 top
GND_3  132.08,3.81 0 top
IC1  50.8,44.45 90 top
IC2  16.51,25.4 90 top
IC2_1  50.8,25.4 90 top
IC2_2  85.09,25.4 90 top
IC2_3  119.38,24.13 90 top
IC3  17.78,46.99 90 top
IC7  90.17,45.09 90 top
IC11  128.27,48.26 90 top
ISO0  23.5,27.94 0 top
ISO1  58.42,27.94 0 top
ISO2  92.08,27.3 0 top
ISO3  125.73,28.57 0 top
J7  128.27,71.12 0 top
PWR  146.69,73.66 0 top
R2  15.88,63.5 270 top
R3  18.41,63.5 90 top
R4_0  20.95,63.5 270 top
R4_1  54.61,63.5 270 top
R4_2  88.9,63.5 270 top
R4_3  129.54,55.88 180 top
R5_0  19.68,54.61 0 top
R5_1  53.34,53.34 0 top
R5_2  88.27,53.34 0 top
R5_3  110.49,53.34 180 top
R6  52.07,63.5 270 top
R6_0  19.68,57.15 180 top
R6_1  53.34,56.52 180 top
R6_2  88.27,55.88 180 top
R6_3  110.49,55.88 0 top
R11  49.53,63.5 90 top
R12  86.36,63.5 270 top
R17  83.82,63.5 270 top
R18  104.14,63.5 270 top
R23  101.6,63.5 270 top
R24  146.69,64.77 270 top
SJ3  15.88,63.5 90 top
SJ4  18.41,63.5 270 top
SJ7  52.07,63.5 90 top
SJ12  49.53,63.5 270 top
SJ13  86.36,63.5 90 top
SJ18  83.82,63.5 90 top
SJ19  104.14,63.5 90 top
SJ24  101.6,63.5 90 top
SPAN0  13.97,85.09 90 top
SPAN1  48.26,85.09 90 top
SPAN2  82.55,85.09 90 top
SPAN3  104.78,85.09 90 top
U$1  31.75,34.29 270 top
U$2  66.04,34.29 270 top
U$3  99.06,33.02 270 top
U$4  133.35,33.02 270 top
ZERO0  21.59,85.09 90 top
ZERO1  55.88,85.09 90 top
ZERO2  90.81,85.09 90 top
ZERO3  112.39,85.09 90 top
ZERO_0  24.13,69.85 0 top
ZERO_1  58.42,68.58 0 top
ZERO_2  93.98,68.58 0 top
ZERO_3  113.03,68.58 0 top

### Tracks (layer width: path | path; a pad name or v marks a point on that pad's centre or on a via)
+12_0
  pour Route15: 1.27,24.13 35.56,24.13 35.56,8.89 1.27,8.89
+12_1
  pour Route15: 36.83,24.13 69.85,24.13 69.85,8.89 36.83,8.89
+12_2
  pour Route15: 71.12,8.89 104.14,8.89 104.14,24.13 71.12,24.13
+12_3
  pour Route15: 109.22,8.89 137.16,8.89 137.16,24.13 109.22,24.13
+12V
  pour Route2: 1.27,87.63 148.59,87.63 147.32,27.94 0,27.94
+12V3  (3 unrouted)
+12V4  (2 unrouted)
+12V10  (2 unrouted)
-12_0
  pour Top: 1.27,24.13 35.56,24.13 35.56,8.89 1.27,8.89
-12_1  (1 unrouted)
  pour Top: 36.83,24.13 69.85,24.13 69.85,8.89 36.83,8.89
-12_2  (1 unrouted)
  pour Top: 71.12,8.89 104.14,8.89 104.14,24.13 71.12,24.13
-12_3
  pour Top: 105.41,8.89 137.16,8.89 137.16,24.13 105.41,24.13
-12V  (30 unrouted)
  Route2 1.016: IC7.4 C9.2@2
  Route15 1.016: ZERO3.A 111.76,87.63 110.49,86.36 110.49,81.28 109.22,80.01 100.33,80.01 96.52,83.82 96.52,86.36 95.25,87.63 ZERO2.A
  pour Top: 1.27,87.63 149.86,87.63 149.86,27.94 1.27,27.94
AIN0+  (1 unrouted)
AIN0_IN  (2 unrouted)
AIN1+  (1 unrouted)
AIN1_IN  (2 unrouted)
AIN2+  (1 unrouted)
AIN2_IN  (2 unrouted)
AIN3+  (1 unrouted)
AIN3_IN  (2 unrouted)
AOUT0  (4 unrouted)
AOUT0+  (1 unrouted)
AOUT0-  (1 unrouted)
AOUT1  (4 unrouted)
AOUT1+  (1 unrouted)
AOUT1-  (1 unrouted)
AOUT2  (4 unrouted)
AOUT2+  (1 unrouted)
AOUT2-  (1 unrouted)
AOUT3  (4 unrouted)
AOUT3+  (1 unrouted)
GND  (59 unrouted)
  pour Route15: 0,87.63 147.32,87.63 147.32,27.94 0,27.94
  pour Bottom: 0,87.63 0,27.94 146.05,27.94 146.05,87.63
GND0
  pour Route2: 1.27,22.86 35.56,22.86 35.56,0 1.27,0
GND0_IN  (2 unrouted)
GND1  (1 unrouted)
  pour Route2: 36.83,24.13 69.85,24.13 69.85,0 36.83,0
GND1_IN  (2 unrouted)
GND2
  pour Route2: 71.12,24.13 104.14,24.13 104.14,0 71.12,0
GND2_IN  (2 unrouted)
GND3
  pour Route2: 105.41,24.13 137.16,24.13 137.16,0 105.41,0
GND3_IN  (2 unrouted)
IC1_9  (3 unrouted)
IC2_8  (3 unrouted)
N$1  (4 unrouted)
N$3  (3 unrouted)
N$4  (3 unrouted)
N$6  (4 unrouted)
N$8  (2 unrouted)
N$17  (3 unrouted)
N$18  (3 unrouted)
N$19  (3 unrouted)
N$22  (2 unrouted)
N$23  (4 unrouted)
N$26  (1 unrouted)
N$27  (3 unrouted)
N$34  (2 unrouted)
N$35  (3 unrouted)
N$36  (3 unrouted)
N$37  (3 unrouted)
N$39  (4 unrouted)
N$40  (4 unrouted)
N$43  (4 unrouted)
N$55  (2 unrouted)
N$56  (4 unrouted)
N$58  (2 unrouted)
N$60  (4 unrouted)
SPAN1L  (2 unrouted)

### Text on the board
Dimension: (150 mm) | (82 mm)
tPlace: Note: ±15V is / also acceptable / for power supply. | - / + | PPISO4: / 4 Channel / Isolation / Amp | 0 1 2 3 | +12 Gnd -12 | Copyright 2020 / Plantation / Productions, Inc. | +Ain0- | +Ain1- | +Ain2- | +Ain3- | 1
